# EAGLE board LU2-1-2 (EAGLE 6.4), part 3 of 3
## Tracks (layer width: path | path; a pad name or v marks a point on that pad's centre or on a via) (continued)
N$406 (continued)
  Bottom 0.305: SV3.7 179.07,90.17 182.25,93.34 186.06,93.34 186.69,93.98 IC37.15
N$407
  Top 0.305: SV3.6 RN26.4
  Bottom 0.305: SV3.6 181.61,90.81 182.88,92.08 191.13,92.08 191.77,92.71 IC37.13
N$408
  Top 0.305: SV3.5 RN26.5
  Bottom 0.305: IC37.11 196.85,94.61 193.68,91.44 184.78,91.44 184.15,90.81 SV3.5
N$409  (via drill 0.6)
  Top 0.305: SV3.4 RN26.6 | IC37.8 191.77,99.69 193.04,98.42 v193.04,87
  Bottom 0.305: v193.04,87 187.96,87 186.69,88.27 SV3.4
N$412
  Top 0.305: RN26.7 SV3.3 189.23,90.81 187.96,92.08 187.96,98.42 186.69,99.69 IC37.6
N$413
  Top 0.305: RN26.8 SV3.2
  Route3 0.305: SV3.2 191.77,92.08 190.5,93.34 190.5,96.52 186.06,100.97 182.25,100.97 181.61,101.6 IC37.4
N$414
  Bottom 0.305: SW16.1 158.75,3.81 154.94,3.81 R37.1
N$415
  Bottom 0.305: SW15.1 129.54,3.81 128.27,5.08 R36.1
N$416
  Bottom 0.305: SW14.1 99.06,3.81 97.79,5.08 R35.1
N$417
  Bottom 0.305: SW13.1 68.58,3.17 67.94,3.81 63.5,3.81 R34.1
N$418
  Bottom 0.305: R33.1 29.21,5.08 SW12.1
N$419
  Top 0.305: S1.16 RN24.9 SV2.1 SV7.1
N$420
  Top 0.305: S1.13 RN24.6 SV2.4 SV7.4
N$421
  Top 0.305: SV10.6 SV8.6 RN8.7 95.25,137.16 95.89,137.79 114.3,137.79 114.94,137.16 114.94,109.86 120.65,104.14 120.65,90.17 121.92,88.9 121.92,84.45 124.46,81.92 124.46,79.38 123.83,78.74 118.75,78.74 118.11,79.38 IC28.13
  Route2 0.305: IC29.7 77.47,76.83 79.38,78.74 106.05,78.74 106.68,79.38 106.68,80.64 107.31,81.28 117.47,81.28 118.11,80.64 IC28.13
N$422  (via drill 0.6)
  Top 0.305: SV10.7 SV8.7 RN8.8 92.71,137.16 93.98,138.43 114.94,138.43 115.57,137.79 115.57,111.76 123.19,104.14 123.19,90.17 124.46,88.9 124.46,83.19 125.09,82.55 v125.73,82.55
  Route2 0.305: IC29.8 81.28,74.93 83.19,74.93 83.82,75.56 83.82,76.83 84.45,77.47 111.76,77.47 113.03,78.74 IC28.15
  Bottom 0.305: IC28.15 113.03,81.28 114.3,82.55 v125.73,82.55
N$423  (via drill 0.6)
  Top 0.305: SV10.8 SV8.8 RN8.9 90.17,137.79 91.44,139.06 115.57,139.06 116.2,138.43 116.2,113.67 125.73,104.14 125.73,90.81 125.41,90.49 v125.41,84.45
  Route2 0.305: IC29.9 82.55,77.47 83.19,78.11 107.31,78.11 107.95,78.74 IC28.17
  Bottom 0.305: IC28.17 107.95,80.64 111.76,84.45 v125.41,84.45
N$424
  Top 0.305: SV10.4 SV8.4 RN8.5 100.33,135.25 101.6,136.53 113.03,136.53 113.67,135.89 113.67,106.05 115.57,104.14 115.57,90.17 IC28.8
  Route2 0.305: IC29.5 72.39,77.47 73.66,78.74 73.66,81.28 74.93,82.55 114.3,82.55 118.11,86.36 IC28.8
N$425
  Top 0.305: SV10.3 SV8.3 RN8.4 102.87,134.62 104.14,135.89 112.39,135.89 113.03,135.25 IC28.6
  Route2 0.305: IC29.4 69.85,77.47 71.12,78.74 71.12,81.28 73.03,83.19 109.86,83.19 113.03,86.36 IC28.6
N$426  (via drill 0.6)
  Top 0.305: SV10.2 SV8.2 RN8.3 105.41,133.99 106.68,135.25 111.76,135.25 112.39,134.62 112.39,106.05 107.95,101.6 IC28.4
  Route2 0.305: IC29.3 67.31,76.83 66.04,78.11 66.04,83.19 v67.31,84.45
  Bottom 0.305: IC28.4 105.41,85.09 69.22,85.09 68.58,84.45 v67.31,84.45
N$427  (via drill 0.6)
  Top 0.305: RN8.2 SV8.1 SV10.1 107.95,125.09 110.49,122.56 110.49,110.49 102.87,102.87 IC28.2
  Route2 0.305: IC29.2 64.77,76.83 63.5,78.11 63.5,82.87 v65.09,84.45
  Bottom 0.305: IC28.2 102.87,87 101.6,85.72 66.36,85.72 v65.09,84.45
N$428  (via drill 0.6)
  Top 0.305: IC32.18 142.24,85.09 140.97,86.36 v140.97,93.98
  Bottom 0.305: v140.97,93.98 137.48,93.98 131.13,100.33 U11.A0
N$429  (via drill 0.6)
  Top 0.305: v146.05,93.66 146.05,85.09 147.32,83.82 IC32.16
  Bottom 0.305: U11.A1 124.46,101.6 125.09,102.23 130.18,102.23 137.16,95.25 144.46,95.25 v146.05,93.66
N$430  (via drill 0.6)
  Top 0.305: v151.13,93.66 151.13,85.09 152.4,83.82 IC32.14
  Bottom 0.305: U11.A2 121.92,102.23 122.56,102.87 131.13,102.87 138.11,95.89 148.91,95.89 v151.13,93.66
N$431  (via drill 0.6)
  Top 0.305: v155.57,93.66 156.21,93.03 156.21,85.09 157.48,83.82 IC32.12
  Bottom 0.305: U11.A3 119.38,102.87 120.02,103.5 132.08,103.5 139.06,96.52 149.86,96.52 150.5,95.89 153.67,95.89 v155.57,93.66
N$432  (via drill 0.6)
  Top 0.305: v157.48,97.79 IC32.9
  Bottom 0.305: U11.A4 116.84,102.87 118.11,104.14 133.03,104.14 140.02,97.16 150.5,97.16 151.13,96.52 156.21,96.52 v157.48,97.79
N$433  (via drill 0.6)
  Top 0.305: IC32.7 v152.4,97.79
  Bottom 0.305: U11.A5 114.3,103.5 115.57,104.78 133.99,104.78 140.97,97.79 v152.4,97.79
N$434  (via drill 0.6)
  Top 0.305: IC32.5 147.32,98.42 147.96,99.06 v147.96,100.33
  Bottom 0.305: U11.A6 111.76,103.5 113.67,105.41 134.94,105.41 140.02,100.33 v147.96,100.33
N$435  (via drill 0.6)
  Top 0.305: IC32.3 142.24,100.97 v139.7,103.5
  Bottom 0.305: U11.A7 109.22,103.5 111.76,106.05 137.16,106.05 v139.7,103.5
N$436
  Top 0.305: RN26.9 SV3.1
  Route3 0.305: SV3.1 194.31,92.71 193.04,93.98 193.04,103.5 192.41,104.14 177.8,104.14 IC37.2
OUTBUSHIGH0  (via drill 0.6)
  Top 0.305: IC2.18 40.64,106.68 | 40.64,106.68 41.27,107.31 v41.27,120.02 | v42.55,95.25 42.55,100.33 41.27,101.6 41.27,106.05 40.64,106.68
  Route2 0.305: P8.32 59.21,96.04 58.42,95.25 v42.55,95.25
  Bottom 0.305: IC1.18 66.67,125.73 65.41,127 55.24,127 51.44,123.19 50.16,123.19 47.62,120.65 41.91,120.65 v41.27,120.02
OUTBUSHIGH1  (via drill 0.6)
  Top 0.305: IC21.19 29.21,60.96 26.67,63.5 IC21.1 26.67,65.41 27.94,66.67 29.84,66.67 30.48,67.31 30.48,76.83 33.02,79.38 v33.02,96.52
  Route2 0.305: P8.33 53.98,99.06 52.7,97.79 34.29,97.79 v33.02,96.52
OUTBUSHIGH2  (via drill 0.6)
  Top 0.305: IC4.19 29.21,71.75 26.67,74.3 IC4.1 26.67,76.83 27.94,78.11 27.94,81.28 24.13,85.09 v24.13,92.71
  Bottom 0.305: P8.34 59.05,99.06 57.78,97.79 53.34,97.79 50.8,95.25 44.45,95.25 41.91,92.71 v24.13,92.71
OUTBUSHIGH3  (via drill 0.6)
  Top 0.305: IC7.19 102.87,71.12 100.33,73.66 IC7.1 100.97,76.2 102.87,78.11 106.05,78.11 106.68,78.74 106.68,84.45 104.14,87 104.14,95.89 v105.41,97.16
  Route3 0.305: P8.35 56.67,101.44 57.78,100.33 60.96,100.33 63.5,97.79 104.78,97.79 v105.41,97.16
OUTBUSHIGH4  (via drill 0.6)
  Top 0.305: IC10.19 139.7,71.75 137.16,74.3 IC10.1 137.16,76.83 138.43,78.11 138.43,81.28 134.62,85.09 134.62,94.61 v130.81,99.06
  Route3 0.305: P8.36 61.59,101.6 62.87,100.33 105.41,100.33 106.68,99.06 v130.81,99.06
OUTBUSHIGH5  (via drill 0.6)
  Top 0.305: IC18.19 173.99,22.23 171.45,24.77 IC18.1 171.45,27.3 173.99,29.84 173.99,55.88 172.72,57.15 172.72,103.19 v172.4,103.5
  Route3 0.305: P8.37 56.67,103.98 57.78,102.87 137.79,102.87 138.43,102.23 166.69,102.23 168.91,104.46 171.45,104.46 v172.4,103.5
OUTBUSHIGH7  (via drill 0.6)
  Top 0.305: IC35.1 177.8,54.61 177.8,106.05 v176.21,107.63
  Route3 0.305: P8.39 57.15,106.68 58.42,105.41 173.99,105.41 v176.21,107.63
  Bottom 0.305: IC35.1 177.8,53.34 175.26,50.8 IC35.19
OUTBUSLOW0  (via drill 0.6)
  Top 0.305: IC15.3 247.65,25.4 246.38,26.67 246.38,30.48 247.65,31.75 IC14.3 247.65,36.2 246.38,37.47 246.38,42.55 247.65,43.81 IC22.3 247.65,48.26 246.38,49.53 246.38,53.34 247.65,54.61 IC13.3 247.65,59.69 246.38,60.96 246.38,64.77 247.65,66.04 IC3.3 247.65,71.12 246.38,72.39 246.38,76.2 247.65,77.47 IC34.3 245.11,83.82 245.11,88.9 246.38,90.17 IC16.3 246.38,93.34 245.11,94.61 245.11,100.33 246.38,101.6 IC17.3 | v206.38,88.9 v206.38,99.69
  Route2 0.305: IC16.3 246.38,92.08 245.75,91.44 242.25,91.44 236.54,85.72 216.53,85.72 213.36,88.9 v206.38,88.9
  Bottom 0.305: P8.42 99.69,96.52 109.86,106.68 138.11,106.68 143.19,101.6 165.1,101.6 167,99.69 v206.38,99.69
OUTBUSLOW1  (via drill 0.6)
  Top 0.305: IC15.4 250.19,25.4 248.92,26.67 248.92,30.48 250.19,31.75 IC14.4 250.19,36.83 248.92,38.1 248.92,42.55 250.19,43.81 IC22.4 250.19,48.26 248.92,49.53 248.92,53.34 250.19,54.61 IC13.4 250.19,59.69 248.92,60.96 248.92,64.77 250.19,66.04 IC3.4 250.19,71.12 248.92,72.39 248.92,76.2 250.19,77.47 IC34.4 250.19,82.55 248.92,83.82 248.28,83.82 247.65,84.45 247.65,88.9 248.92,90.17 IC16.4 248.92,93.98 247.65,95.25 247.65,100.33 248.92,101.6 IC17.4 | v203.84,101.6 v203.84,87
  Route2 0.305: IC16.4 248.92,91.44 248.28,90.81 242.57,90.81 236.85,85.09 215.9,85.09 214,87 v203.84,87
  Bottom 0.305: P8.43 87,99.06 88.27,100.33 100.97,100.33 108.58,107.95 138.75,107.95 141.92,104.78 141.86,104.78 143.76,102.87 166.37,102.87 168.28,100.97 203.2,100.97 v203.84,101.6
OUTBUSLOW2  (via drill 0.6)
  Top 0.305: IC15.7 257.81,25.4 256.54,26.67 256.54,30.48 257.81,31.75 IC14.7 257.81,36.2 256.54,37.47 256.54,42.55 257.81,43.81 IC22.7 257.81,48.26 256.54,49.53 256.54,53.34 257.81,54.61 IC13.7 257.81,59.69 256.54,60.96 256.54,64.77 257.81,66.04 IC3.7 257.81,71.12 256.54,72.39 256.54,76.2 257.81,77.47 IC34.7 255.27,83.82 255.27,88.9 256.54,90.17 IC16.7 256.54,94.61 255.27,95.89 255.27,97.79 256.54,99.06 IC17.7 | v205.1,100.97 v205.1,85.72
  Route2 0.305: IC16.7 256.54,91.44 255.27,90.17 242.89,90.17 237.17,84.45 215.26,84.45 214,85.72 v205.1,85.72
  Bottom 0.305: P8.44 100.97,99.06 109.22,107.31 138.43,107.31 143.51,102.23 165.74,102.23 167.64,100.33 204.47,100.33 v205.1,100.97
OUTBUSLOW3  (via drill 0.6)
  Top 0.305: IC15.8 260.35,25.4 259.08,26.67 259.08,30.48 260.35,31.75 IC14.8 260.35,36.83 259.08,38.1 259.08,42.55 260.35,43.81 IC22.8 260.35,48.26 259.08,49.53 259.08,53.34 260.35,54.61 IC13.8 260.35,59.69 259.08,60.96 259.08,64.77 260.35,66.04 IC3.8 260.35,71.12 259.08,72.39 259.08,76.2 260.35,77.47 IC34.8 260.35,82.55 259.08,83.82 258.44,83.82 257.81,84.45 257.81,88.27 259.08,89.53 IC16.8 259.08,94.61 257.81,95.89 257.81,100.33 259.08,101.6 IC17.8
  Route2 0.305: IC17.8 259.08,103.5 258.44,102.87 212.72,102.87 208.91,106.68 180.97,106.68 177.8,109.86 v173.99,109.86
  Bottom 0.305: P8.45 87.31,101.6 88.58,102.87 100.97,102.87 107.31,109.22 139.38,109.22 142.56,106.05 168.59,106.05 172.4,109.86 v173.99,109.86
OUTBUSLOW4  (via drill 0.6)
  Top 0.305: IC15.13 260.35,19.68 261.62,20.95 261.62,25.4 260.35,26.67 IC14.13 260.35,30.48 261.62,31.75 261.62,36.83 260.35,38.1 IC22.13 260.35,42.55 261.62,43.81 261.62,48.26 260.35,49.53 IC13.13 260.35,53.34 261.62,54.61 261.62,59.69 260.35,60.96 IC3.13 260.35,64.77 261.62,66.04 261.62,71.12 260.35,72.39 IC34.13 260.35,76.2 261.62,77.47 261.62,82.55 IC16.13 259.08,88.27 260.35,89.53 260.35,94.61 259.08,95.89 IC17.13
  Route2 0.305: IC17.13 256.54,99.06 254,99.06 252.09,100.97 241.3,100.97 240.66,101.6 212.09,101.6 208.28,105.41 179.71,105.41 178.44,106.68 v173.35,106.68
  Bottom 0.305: P8.46 100.97,101.6 107.95,108.58 139.06,108.58 142.24,105.41 168.91,105.41 170.18,106.68 v173.35,106.68
OUTBUSLOW5  (via drill 0.6)
  Top 0.305: IC15.14 257.81,19.68 259.08,20.95 259.08,25.4 257.81,26.67 IC14.14 257.81,30.48 259.08,31.75 259.08,36.83 257.81,38.1 IC22.14 257.81,42.55 259.08,43.81 259.08,48.26 257.81,49.53 IC13.14 257.81,53.34 259.08,54.61 259.08,59.69 257.81,60.96 IC3.14 257.81,64.77 259.08,66.04 259.08,71.12 257.81,72.39 IC34.14 257.81,76.2 259.08,77.47 259.08,82.55 258.44,83.19 257.18,83.19 256.54,83.82 IC16.14 256.54,88.9 257.81,90.17 257.81,94.61 256.54,95.89 IC17.14
  Route2 0.305: IC17.14 254.63,98.42 248.92,98.42 248.28,99.06 241.94,99.06 240.03,100.97 211.77,100.97 207.96,104.78 179.07,104.78 178.44,105.41 171.13,105.41 169.23,107.31 v169.23,109.22
  Bottom 0.305: P8.47 86.67,104.45 87.63,105.41 100.97,105.41 106.05,110.49 140.02,110.49 143.19,107.31 167.32,107.31 v169.23,109.22
OUTBUSLOW6  (via drill 0.6)
  Top 0.305: IC15.17 250.19,19.68 251.46,20.95 251.46,25.4 250.19,26.67 IC14.17 250.19,30.48 251.46,31.75 251.46,36.83 250.19,38.1 IC22.17 250.19,42.55 251.46,43.81 251.46,48.26 250.19,49.53 IC13.17 250.19,53.34 251.46,54.61 251.46,59.69 250.19,60.96 IC3.17 250.19,64.77 251.46,66.04 251.46,71.12 250.19,72.39 IC34.17 250.19,76.2 251.46,77.47 251.46,82.55 IC16.17 248.92,88.9 250.19,90.17 250.19,93.98 248.92,95.25 IC17.17 | v212.72,118.11 213.36,117.47 213.36,84.45 v214,83.82
  Route2 0.305: IC16.17 248.92,86.36 248.28,87 240.66,87 237.49,83.82 v214,83.82
  Bottom 0.305: P8.48 100.97,104.14 106.68,109.86 139.7,109.86 142.88,106.68 168.28,106.68 173.99,112.39 203.84,112.39 205.74,114.3 208.91,114.3 v212.72,118.11
OUTBUSLOW7  (via drill 0.6)
  Top 0.305: IC15.18 247.65,19.68 248.92,20.95 248.92,25.4 247.65,26.67 IC14.18 247.65,30.48 248.92,31.75 248.92,36.83 247.65,38.1 IC22.18 247.65,42.55 248.92,43.81 248.92,48.26 247.65,49.53 IC13.18 247.65,53.34 248.92,54.61 248.92,59.69 247.65,60.96 IC3.18 247.65,64.77 248.92,66.04 248.92,71.12 247.65,72.39 IC34.18 247.65,76.2 248.92,77.47 248.92,82.55 248.28,83.19 247.01,83.19 246.38,83.82 IC16.18 246.38,88.9 247.65,90.17 247.65,93.34 246.38,94.61 IC17.18
  Route2 0.305: IC17.18 246.38,97.16 245.75,97.79 214,97.79 207.65,104.14 178.44,104.14 177.8,104.78 170.18,104.78 167.64,107.31 v167.64,109.22
  Bottom 0.305: P8.49 86.67,108.26 89.53,111.12 140.34,111.12 143.51,107.95 166.37,107.95 v167.64,109.22
OUTBUSLOW8
  Top 0.305: IC21.18 31.75,35.56 SV6.1
  Bottom 0.305: SV6.1 SV5.1
OUTBUSLOW9
  Route2 0.305: IC21.16 36.83,55.88 36.2,55.24 33.66,55.24 33.02,54.61 33.02,46.99 31.75,45.72 29.84,45.72 29.21,45.09 29.21,38.1 SV6.2
  Bottom 0.305: SV5.2 SV6.2
OUTBUSLOW10
  Route2 0.305: SV6.3 33.02,39.37 34.29,40.64 36.83,40.64 37.47,41.27 37.47,51.44 41.91,55.88 IC21.14
  Bottom 0.305: SV6.3 SV5.3
OUTBUSLOW11
  Route2 0.305: SV6.4 33.02,41.91 34.29,43.18 34.29,53.34 34.92,53.98 38.73,53.98 40.64,55.88 40.64,57.78 41.27,58.42 46.35,58.42 46.99,57.78 IC21.12
  Bottom 0.305: SV6.4 SV5.4
OUTBUSLOW12
  Route2 0.305: SV6.5 32.38,44.45 33.66,45.72 33.66,53.98 34.29,54.61 36.83,54.61 38.1,55.88 38.1,58.42 41.91,62.23 46.35,62.23 46.99,62.87 IC21.9
  Bottom 0.305: SV6.5 SV5.5
OUTBUSLOW13
  Route2 0.305: SV6.6 32.38,48.9 32.38,54.93 33.34,55.88 34.92,55.88 35.56,56.52 35.56,59.05 39.37,62.87 41.27,62.87 41.91,63.5 IC21.7
  Bottom 0.305: SV6.6 SV5.6
OUTBUSLOW14
  Route2 0.305: SV6.7 31.11,49.53 31.75,50.16 31.75,55.24 33.02,56.52 33.02,59.69 36.83,63.5 IC21.5
  Bottom 0.305: SV6.7 SV5.7
OUTBUSLOW15
  Top 0.305: IC21.3 31.75,62.23 30.48,60.96 SV6.8
  Bottom 0.305: SV6.8 SV5.8
VCC  (via drill 0.6)
  Top 0.813: C8.1 198.12,6.35 R38.2
  Top 1.016: IC26.20 62.23,81.28 62.87,81.92 62.87,85.41 62.23,86.04 IC26.1 | C34.1 53.34,83.82 51.44,85.72 v51.44,91.44 | C14.1 88.9,67.94 90.81,66.04 90.81,64.45 88.9,62.55 C13.1 | IC13.20 241.94,50.8 | 240.66,61.59 241.3,62.23 | 240.66,73.03 241.3,73.66 IC34.20 | IC8.20 102.87,52.07 105.41,49.53 v105.41,27.3 105.41,25.4 104.14,24.13 v104.14,5.08 | IC37.20 v173.99,98.74
  Top 1.27: IC30.20 151.13,134.62 RN23.1 IC31.1 IC31.20 | C28.1 269.88,16.51 271.14,17.78 271.14,26.04 C29.1 271.14,29.84 271.14,37.47 C30.1 271.14,41.27 271.14,48.9 C31.1 271.14,52.7 271.14,60.33 C32.1 271.14,64.14 271.14,71.75 C4.1 271.14,75.56 271.14,83.82 269.88,85.09 C7.1 | 165.1,68.58 165.74,69.22 165.74,78.11 C37.1 v163.83,85.09 | C17.1 165.1,68.58 | 165.1,68.58 165.74,67.94 165.74,62.87 163.83,60.96 C38.1 | IC9.20 137.16,55.24 138.43,53.98 IC11.20 | IC37.20 RN26.1 | C42.1 207.01,39.37 205.74,40.64 C11.1 | IC23.2 48.26,140.97 48.9,140.34 48.9,136.53 48.26,135.89 | IC23.4 48.26,135.89 | 48.26,135.89 48.9,135.25 48.9,126.36 47.62,125.09 C19.1
  Top 1.422: P8.19 23.11,138.68 19.05,134.62 C5.1 21.59,113.03 21.59,97.16 19.05,94.61 C3.+ 20.32,92.71 21.59,91.44 21.59,85.09 IC5.20 24.77,78.11 24.77,70.48 IC4.20 | IC1.24 66.04,140.97 64.77,139.7 RN2.1 | IC26.20 IC29.1 IC29.20 IC27.1 IC27.20 | C6.1 179.07,134.62 RN24.1 179.07,110.49 IC24.20 | R18.2 206.38,123.83 206.38,114.3 v207.65,113.03 208.28,112.39 C26.1 v208.28,95.25 | IC25.20 C10.1 | v179.07,55.24 IC12.20 | 241.3,27.94 240.66,27.3 v240.66,22.86 240.66,18.41 IC15.20 | IC14.20 241.3,27.94 | 241.3,27.94 240.66,28.57 240.66,38.73 241.3,39.37 | IC22.20 241.3,39.37 | 241.3,39.37 240.66,40.01 240.66,50.16 241.3,50.8 IC13.20 | 241.94,50.8 240.66,52.07 240.66,61.59 | IC3.20 241.3,62.23 240.66,62.87 240.66,73.03 | 241.3,73.66 240.66,74.3 240.66,82.55 241.3,83.19 IC16.20 241.3,90.17 239.4,92.08 239.4,92.71 238.12,93.98 U16.8 | v171.45,5.08 IC19.20 170.81,8.89 169.54,10.16 169.54,18.41 170.18,19.05 | 170.18,19.05 IC18.20 | C8.1 196.22,10.79 196.22,17.78 197.49,19.05 C9.1 | IC2.24 37.47,121.92 35.56,120.02 RN4.1 | v46.99,6.35 45.09,8.26 v45.21,25.84 48.26,29.21 RN11.1 | IC7.20 100.33,70.48 98.42,72.39 98.42,78.11 IC28.20 | IC6.20 100.33,55.88 101.6,54.61 IC8.20 | C15.1 127,54.61 126.36,53.98 126.36,32.38 128.27,30.48 C45.1 | C43.1 168.28,27.3 168.91,26.67 168.91,20.32 170.18,19.05 | 246.38,121.92 R14.2 245.11,125.73 243.21,123.83 239.4,123.83 237.49,125.73 R16.2 | 246.38,121.92 v246.38,109.86 | IC20.20 C38.1 | IC32.20 135.89,80.01 135.25,79.38 135.25,73.66 137.16,71.75 IC10.20 | IC26.1 62.23,100.33 v63.5,101.6 | R1.2 246.38,121.92
  Route2 0.508: v46.99,6.35 53.34,6.35 54.61,5.08 R22.2 59.69,5.08 60.96,6.35 63.5,6.35 64.77,5.08 R34.2 76.83,5.08 78.11,6.35 83.82,6.35 85.09,5.08 R21.2 | R35.2 v104.14,5.08 106.68,5.08 107.95,6.35 114.94,6.35 116.2,5.08 R20.2 120.65,5.08 121.92,6.35 129.54,6.35 R36.2
  Route2 0.61: R19.2 146.05,5.08 145.1,4.13 141.92,4.13 141.6,3.81 140.97,3.81 139.7,2.54
  Route2 1.016: R36.2 133.35,2.54 139.7,2.54
  Route2 1.27: C42.1 207.65,37.47 215.9,37.47 | 215.9,37.47 222.88,37.47 224.79,39.37 IC22.20 | RN23.1 153.67,132.72 154.94,133.99 178.44,133.99 179.07,133.35 RN24.1 | v240.66,111.76 241.94,111.76 243.84,109.86 v246.38,109.86 | IC34.20 245.11,76.2 265.43,76.2 267.97,73.66 C4.1 | 215.9,37.47 215.9,24.13 217.17,22.86 U13.3 | IC6.20 99.06,57.15 98.42,57.78 98.42,67.94 99.06,68.58 IC7.20
  Route2 1.422: v51.44,91.44 60.96,91.44 62.23,90.17 IC26.1 | RN22.1 RN11.1 | RN10.1 17.78,54.61 | 17.78,54.61 17.78,68.58 | IC21.20 26.67,55.88 25.4,54.61 17.78,54.61 | C5.1 19.05,118.11 22.86,121.92 IC2.24 | C29.1 269.24,28.57 267.97,29.84 243.21,29.84 242.57,29.21 IC14.20 | R1.2 248.92,120.65 215.9,120.65 210.82,125.73 R18.2 | C17.1 172.09,68.58 175.26,71.75 198.12,71.75 199.39,73.03 206.38,73.03 207.01,72.39 v210.19,72.39 211.46,73.66 IC34.20
  Route2 1.676: U1.D 10.16,71.12 12.7,68.58 17.78,68.58 IC4.20
  Route3 0.508: R21.2 89.53,5.08 90.81,6.35 99.06,6.35 R35.2
  Route3 1.016: IC32.20 137.16,78.74 137.79,78.11 163.19,78.11 163.83,78.74 C37.1
  Route3 1.27: C25.1 200.66,87.63 210.19,78.11 v210.19,72.39 210.19,71.75 208.28,69.85 208.28,60.96 207.01,59.69 C11.1 | IC22.20 242.57,40.64 243.84,41.91 267.97,41.91 269.24,40.64 C30.1 | U16.8 238.12,93.98 239.4,95.25 239.4,110.49 v240.66,111.76 | RN11.1 50.16,33.66 50.16,53.98 C33.1
  Route3 1.422: C15.1 127,60.96 125.09,62.87 125.09,66.67 C36.1 | IC20.20 163.19,53.34 165.1,51.44 165.1,29.21 167,27.3 C43.1 | IC25.20 197.49,53.34 200.03,50.8 200.03,20.95 C9.1 | v85.72,31.75 85.72,52.7 88.9,55.88 C13.1 | RN8.1 v118.75,133.35 | IC19.20 171.45,10.16 172.72,11.43 197.49,11.43 198.12,10.79 C8.1 | RN24.1 179.07,130.18 181.61,127.64 200.66,127.64 202.56,125.73 R18.2
  Bottom 0.508: R21.2 85.09,5.08 83.82,6.35 78.11,6.35 76.83,5.08 R34.2 64.77,5.08 63.5,6.35 60.96,6.35 59.69,5.08 R22.2 54.61,5.08 53.34,6.35 v46.99,6.35 | 89.53,5.08 90.81,6.35 99.06,6.35 R35.2 v104.14,5.08 106.68,5.08 107.95,6.35 114.94,6.35 116.2,5.08 R20.2 120.65,5.08 121.92,6.35 129.54,6.35 R36.2
  Bottom 0.61: R21.2 89.53,5.08 | R19.2 149.86,5.08 151.13,6.35 154.31,6.35 155.57,5.08 R37.2 | R18.2 208.28,125.09 209.55,123.83 216.53,123.83 218.44,125.73 R17.2 226.69,125.73 227.97,127 232.41,127 R16.2
  Bottom 0.813: C8.1 197.49,8.89 194.63,6.03 R8.2
  Bottom 1.016: C34.1 IC26.20 | C10.1 200.66,56.52 202.25,58.1 204.15,58.1 C11.1 | v173.99,98.74 199.71,98.74 200.66,97.79 C25.1 | C45.1 129.54,29.21 RN12.1 136.21,27.62 148.59,27.62 149.86,28.89 162.56,28.89 164.15,27.3 C43.1 | IC30.20 145.41,135.89 142.56,133.03 119.06,133.03 v118.75,133.35 | v246.38,109.86 255.91,109.86 256.54,109.22 C41.1
  Bottom 1.27: C27.1 IC31.1 | IC10.20 C36.1 | C15.1 IC9.20 137.16,59.05 137.79,59.69 161.93,59.69 163.83,57.78 C38.1 | IC24.20 181.61,109.22 183.51,111.12 205.74,111.12 v207.65,113.03 | 48.9,140.97 49.53,141.6 64.14,141.6 64.77,140.97 | C12.1 50.8,71.12 27.3,71.12 26.67,70.48 IC4.20
  Bottom 1.422: IC2.24 42.55,121.92 45.72,125.09 C19.1 50.16,125.09 RN3.1 | P8.19 P8.20 30.09,138.68 34.92,143.51 IC23.14 41.91,143.51 44.45,140.97 IC23.2 48.9,140.97 | C14.1 IC7.20 100.33,69.85 100.97,70.48 125.73,70.48 127,69.22 C36.1 | 100.33,58.42 99.69,59.05 90.81,59.05 C13.1 87,59.05 62.87,59.05 62.23,58.42 IC27.20 C33.1 50.8,54.61 39.37,54.61 36.83,52.07 IC33.20 33.66,53.98 27.94,53.98 26.67,55.24 IC21.20 | C35.1 88.9,81.28 | 88.9,81.28 89.53,81.92 99.69,81.92 100.33,81.28 IC28.20 | C16.1 IC32.20 | C12.1 IC29.20 | RN10.1 17.78,25.4 18.41,26.04 28.31,26.04 arc45 28.76,26.22 30.48,27.94 | v45.21,25.84 32.84,25.84 arc-45 32.39,26.03 30.48,27.94 | 30.48,27.94 C39.1 | RN22.1 v85.72,31.75 95.25,31.75 C24.1 99.69,27.3 v105.41,27.3 | IC25.20 191.13,53.34 189.87,54.61 RN9.1 184.78,54.61 184.15,55.24 v179.07,55.24 176.53,55.24 174.62,53.34 IC35.20 171.45,54.61 170.81,55.24 165.74,55.24 163.83,53.34 IC20.20 | IC17.20 240.03,95.25 239.4,95.25 238.12,93.98 U16.8 U16.3 U15.8 U15.3 217.81,93.98 216.53,95.25 v208.28,95.25 C25.1 | v240.66,22.86 U14.8 U14.3 U13.8 U13.3 214,22.86 210.19,19.05 C9.1 198.12,20.32 196.85,21.59 172.09,21.59 171.45,20.95 IC18.20 | R37.2 v171.45,5.08 | R4.2 C41.1 | C7.1 269.24,86.36 268.61,87 241.94,87 241.3,86.36 IC16.20 | IC15.20 242.57,18.41 243.21,19.05 268.61,19.05 269.24,18.41 C28.1 | 64.77,140.97 IC1.24 67.31,142.24 68.58,143.51 RN1.1 81.28,143.51 86.36,138.43 116.2,138.43 118.75,135.89 v118.75,133.35 | R33.2 45.72,5.08 v46.99,6.35 | 88.9,81.28 88.27,81.92 62.87,81.92 62.23,81.28 IC26.20 | C15.1 127,58.42 126.36,59.05 100.97,59.05 100.33,58.42
  Bottom 1.422: 100.33,58.42 IC6.20 | RN26.1 172.72,85.09 v163.83,85.09 | C18.1 v51.44,91.44 | C20.1 v63.5,101.6
  pour Route2: 19.68,27.94 1.91,27.94 arc-90 1.27,28.57 1.27,70.48 arc-90 1.91,71.12 19.68,71.12 arc-90 20.32,70.48 20.32,28.57 arc-90

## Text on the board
Top: LU2 | v2.0 | 2019-04-08
Bottom: v2.0 | 2019-04-08 | LU2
